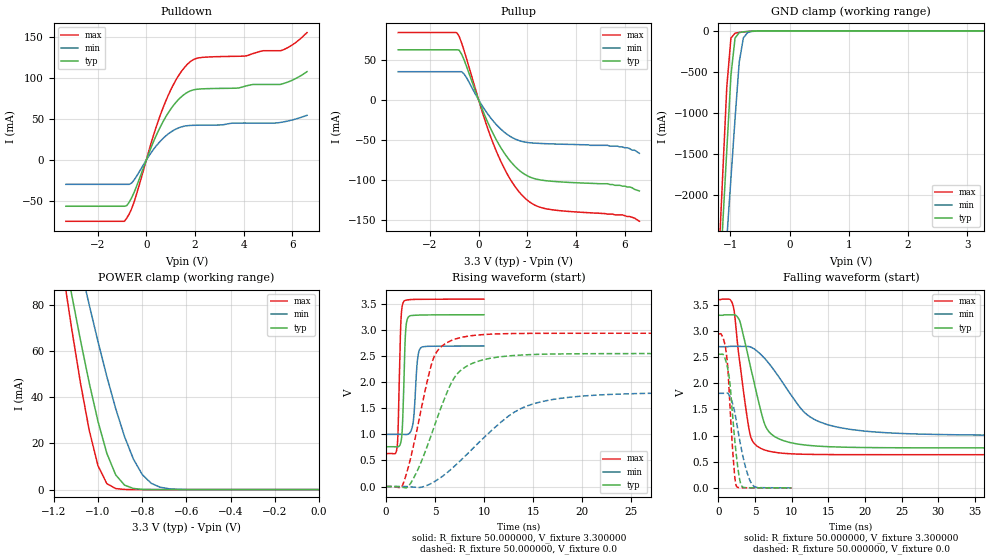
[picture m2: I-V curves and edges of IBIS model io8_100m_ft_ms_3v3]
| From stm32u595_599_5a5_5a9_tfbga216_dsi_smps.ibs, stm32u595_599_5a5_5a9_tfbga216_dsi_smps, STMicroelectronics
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|   Model io8_100m_ft_ms_3v3
[Model]  io8_100m_ft_ms_3v3
Model_type I/O
Polarity   Non-Inverting
Enable   Active-Low
Vinl =   0.990000V
Vinh =   2.310000V
Vmeas =  1.650000V
Cref =   50.000000pF
Rref =   100.000000M
Vref =   0.0V
C_comp   3.313100pF   3.281800pF   3.354500pF
[Temperature Range]   25.000000   0.140000k   -40.000000
[Pullup Reference]   3.300000V   2.700000V   3.600000V
[Pulldown Reference]   0.0V   0.0V   0.0V
[POWER Clamp Reference]   3.300000V   2.700000V   3.600000V
[GND Clamp Reference]   0.0V   0.0V   0.0V
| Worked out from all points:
|   slope of the pulldown table from 0 to 0.495 V, typ, clamps not added: 14 ohm
|   slope of the pullup table from 0 to 0.495 V, typ, clamps not added: 13.7 ohm
|   GND clamp passes 1 mA (typ) near -0.51 V on its own axis
|   POWER clamp passes 1 mA (typ) near -0.85 V on its own axis
|   rising waveform, R_fixture 50.000000, V_fixture 3.300000: 20-80 % time 250ps typ, 341ps min, 235ps max; typ from 0.764 V to 3.3 V
|   rising waveform, R_fixture 50.000000, V_fixture 0.0: 20-80 % time 3.15ns typ, 6.44ns min, 2.09ns max; typ from 0 V to 2.55 V
|   falling waveform, R_fixture 50.000000, V_fixture 3.300000: 20-80 % time 2.58ns typ, 5.7ns min, 1.62ns max; typ from 3.3 V to 0.764 V
|   falling waveform, R_fixture 50.000000, V_fixture 0.0: 20-80 % time 1ns typ, 1.54ns min, 767ps max; typ from 2.55 V to 0 V
[Pulldown]
|Voltage   I(typ)   I(min)   I(max)
-3.3V     -56.06mA   -29.42mA   -74.35mA
-900mV    -56.06mA   -29.42mA   -74.35mA
-700mV    -51.09mA   -29.42mA   -65.48mA
-500mV    -39.32mA   -24.2mA    -50.88mA
300mV     22.62mA    13.13mA    30.43mA
800mV     52.54mA    29.36mA    71.75mA
1.3V      72.91mA    38.82mA    101.4mA
1.8V      84.02mA    42.13mA    119.4mA
2.2V      86.43mA    42.46mA    124.5mA
5.5V      91.98mA    45.75mA    132.9mA
6.1V      98.6mA     49.6mA     142.1mA
6.6V      107.5mA    54.5mA     155mA
[Pullup]
|Voltage   I(typ)   I(min)   I(max)
-3.3V     62.56mA    35.13mA    84.08mA
-900mV    62.56mA    35.13mA    84.08mA
-800mV    62.09mA    35.13mA    79.52mA
-600mV    50.26mA    32.46mA    61.94mA
200mV     -15.65mA   -9.933mA   -19.95mA
700mV     -48.51mA   -30.11mA   -62.22mA
1.3V      -76.68mA   -45.83mA   -99.4mA
2V        -95.1mA    -53.38mA   -125.6mA
2.9V      -101.6mA   -55.08mA   -137mA
5.7V      -107mA     -58mA      -144mA
6.2V      -109mA     -61mA      -146mA
6.6V      -114mA     -67mA      -152mA
[GND_clamp]
|Voltage   I(typ)   I(min)   I(max)
-3.3V     -9.848A    -9.957A    -9.458A
-1.2V     -3.312A    -4.013A    -2.863A
-1.13V    -2.381A    -3.274A    -1.769A
-1.06V    -1.452A    -2.535A    -684.7mA
-990mV    -542.9mA   -1.798A    -88.02mA
-920mV    -87.11mA   -1.064A    -28.44mA
-850mV    -22.1mA    -382.4mA   -19.61mA
-780mV    -11.97mA   -86.98mA   -13.71mA
-710mV    -7.619mA   -22.26mA   -8.745mA
-640mV    -4.493mA   -7.773mA   -4.817mA
-360mV    -31.22uA   -172.6uA   -8.607uA
3.28V     0A         15.66nA    -5.841nA
[POWER_clamp]
|Voltage   I(typ)   I(min)   I(max)
-3.28V    1.355A     1.167A     1.664A
-1.16V    105.7mA    131.6mA    95.69mA
-1.12V    84.97mA    114mA      70.27mA
-1.08V    65.05mA    96.83mA    46.54mA
-1.04V    46.34mA    80.15mA    25.76mA
-1V       29.51mA    64.13mA    10.3mA
-960mV    15.69mA    48.99mA    2.571mA
-920mV    6.373mA    35.1mA     455.6uA
-840mV    490.7uA    13.24mA    11.36uA
-760mV    27.33uA    2.767mA    276.6nA
-640mV    346.6nA    134.1uA    15.62nA
0V        0A         19.91nA    0A
[Ramp]
| variable   typ   min   max
dV/dt_r  1.53252/3.14533n   1.08432/6.43641n   1.76664/2.08469n
dV/dt_f  1.52149/2.57144n   1.01880/5.68990n   1.77964/1.61689n
R_load = 50.000000
[Rising Waveform]
R_fixture= 50.000000
V_fixture= 3.300000
V_fixture_min= 2.700000
V_fixture_max= 3.600000
|time   V(typ)   V(min)   V(max)
0s        764.2mV    1.002V     633.9mV
1.121ns   761.3mV    1.002V     757.3mV
1.502ns   853.5mV    1.002V     3.155V
1.782ns   1.819V     1.001V     3.55V
1.982ns   2.969V     999.4mV    3.578V
2.262ns   3.256V     1.007V     3.587V
2.763ns   3.288V     1.245V     3.594V
3.183ns   3.292V     2.408V     3.595V
3.483ns   3.294V     2.654V     3.596V
9.97ns    3.3V       2.7V       3.6V
[Rising Waveform]
R_fixture= 50.000000
V_fixture= 0.0
V_fixture_min= 0.0
V_fixture_max= 0.0
|time   V(typ)   V(min)   V(max)
0s        9.55uV     6.879uV    8.864uV
1.562ns   -13.37mV   62.23uV    -14.31mV
2.523ns   70.26mV    -6.955mV   566.2mV
4.805ns   1.098V     80.22mV    2.452V
6.366ns   1.877V     289.8mV    2.779V
7.327ns   2.18V      452.1mV    2.848V
9.489ns   2.413V     851.5mV    2.913V
13.09ns   2.517V     1.43V      2.939V
17.66ns   2.547V     1.691V     2.944V
59.82ns   2.554V     1.807V     2.944V
[Falling Waveform]
R_fixture= 50.000000
V_fixture= 3.300000
V_fixture_min= 2.700000
V_fixture_max= 3.600000
|time   V(typ)   V(min)   V(max)
0s        3.3V       2.7V       3.6V
1.922ns   3.308V     2.706V     3.516V
2.162ns   3.307V     2.706V     3.364V
2.883ns   3.198V     2.706V     2.423V
4.324ns   2.34V      2.696V     1.016V
6.366ns   1.196V     2.465V     720.8mV
8.168ns   941.8mV    2.135V     670.7mV
11.77ns   820.2mV    1.439V     642.4mV
16.22ns   781.8mV    1.161V     635.7mV
59.82ns   764.2mV    1.002V     633.9mV
[Falling Waveform]
R_fixture= 50.000000
V_fixture= 0.0
V_fixture_min= 0.0
V_fixture_max= 0.0
|time   V(typ)   V(min)   V(max)
0s        2.554V     1.807V     2.944V
640.6ps   2.549V     1.807V     2.86V
1.101ns   2.377V     1.809V     2.536V
1.281ns   2.262V     1.808V     2.27V
1.542ns   2.023V     1.751V     1.63V
2.042ns   1.194V     1.554V     512.9mV
2.442ns   615.6mV    1.273V     35.5mV
3.123ns   46.74mV    742.7mV    2.616mV
4.625ns   1.603mV    57.94mV    887.5uV
9.97ns    9.55uV     6.879uV    8.864uV
